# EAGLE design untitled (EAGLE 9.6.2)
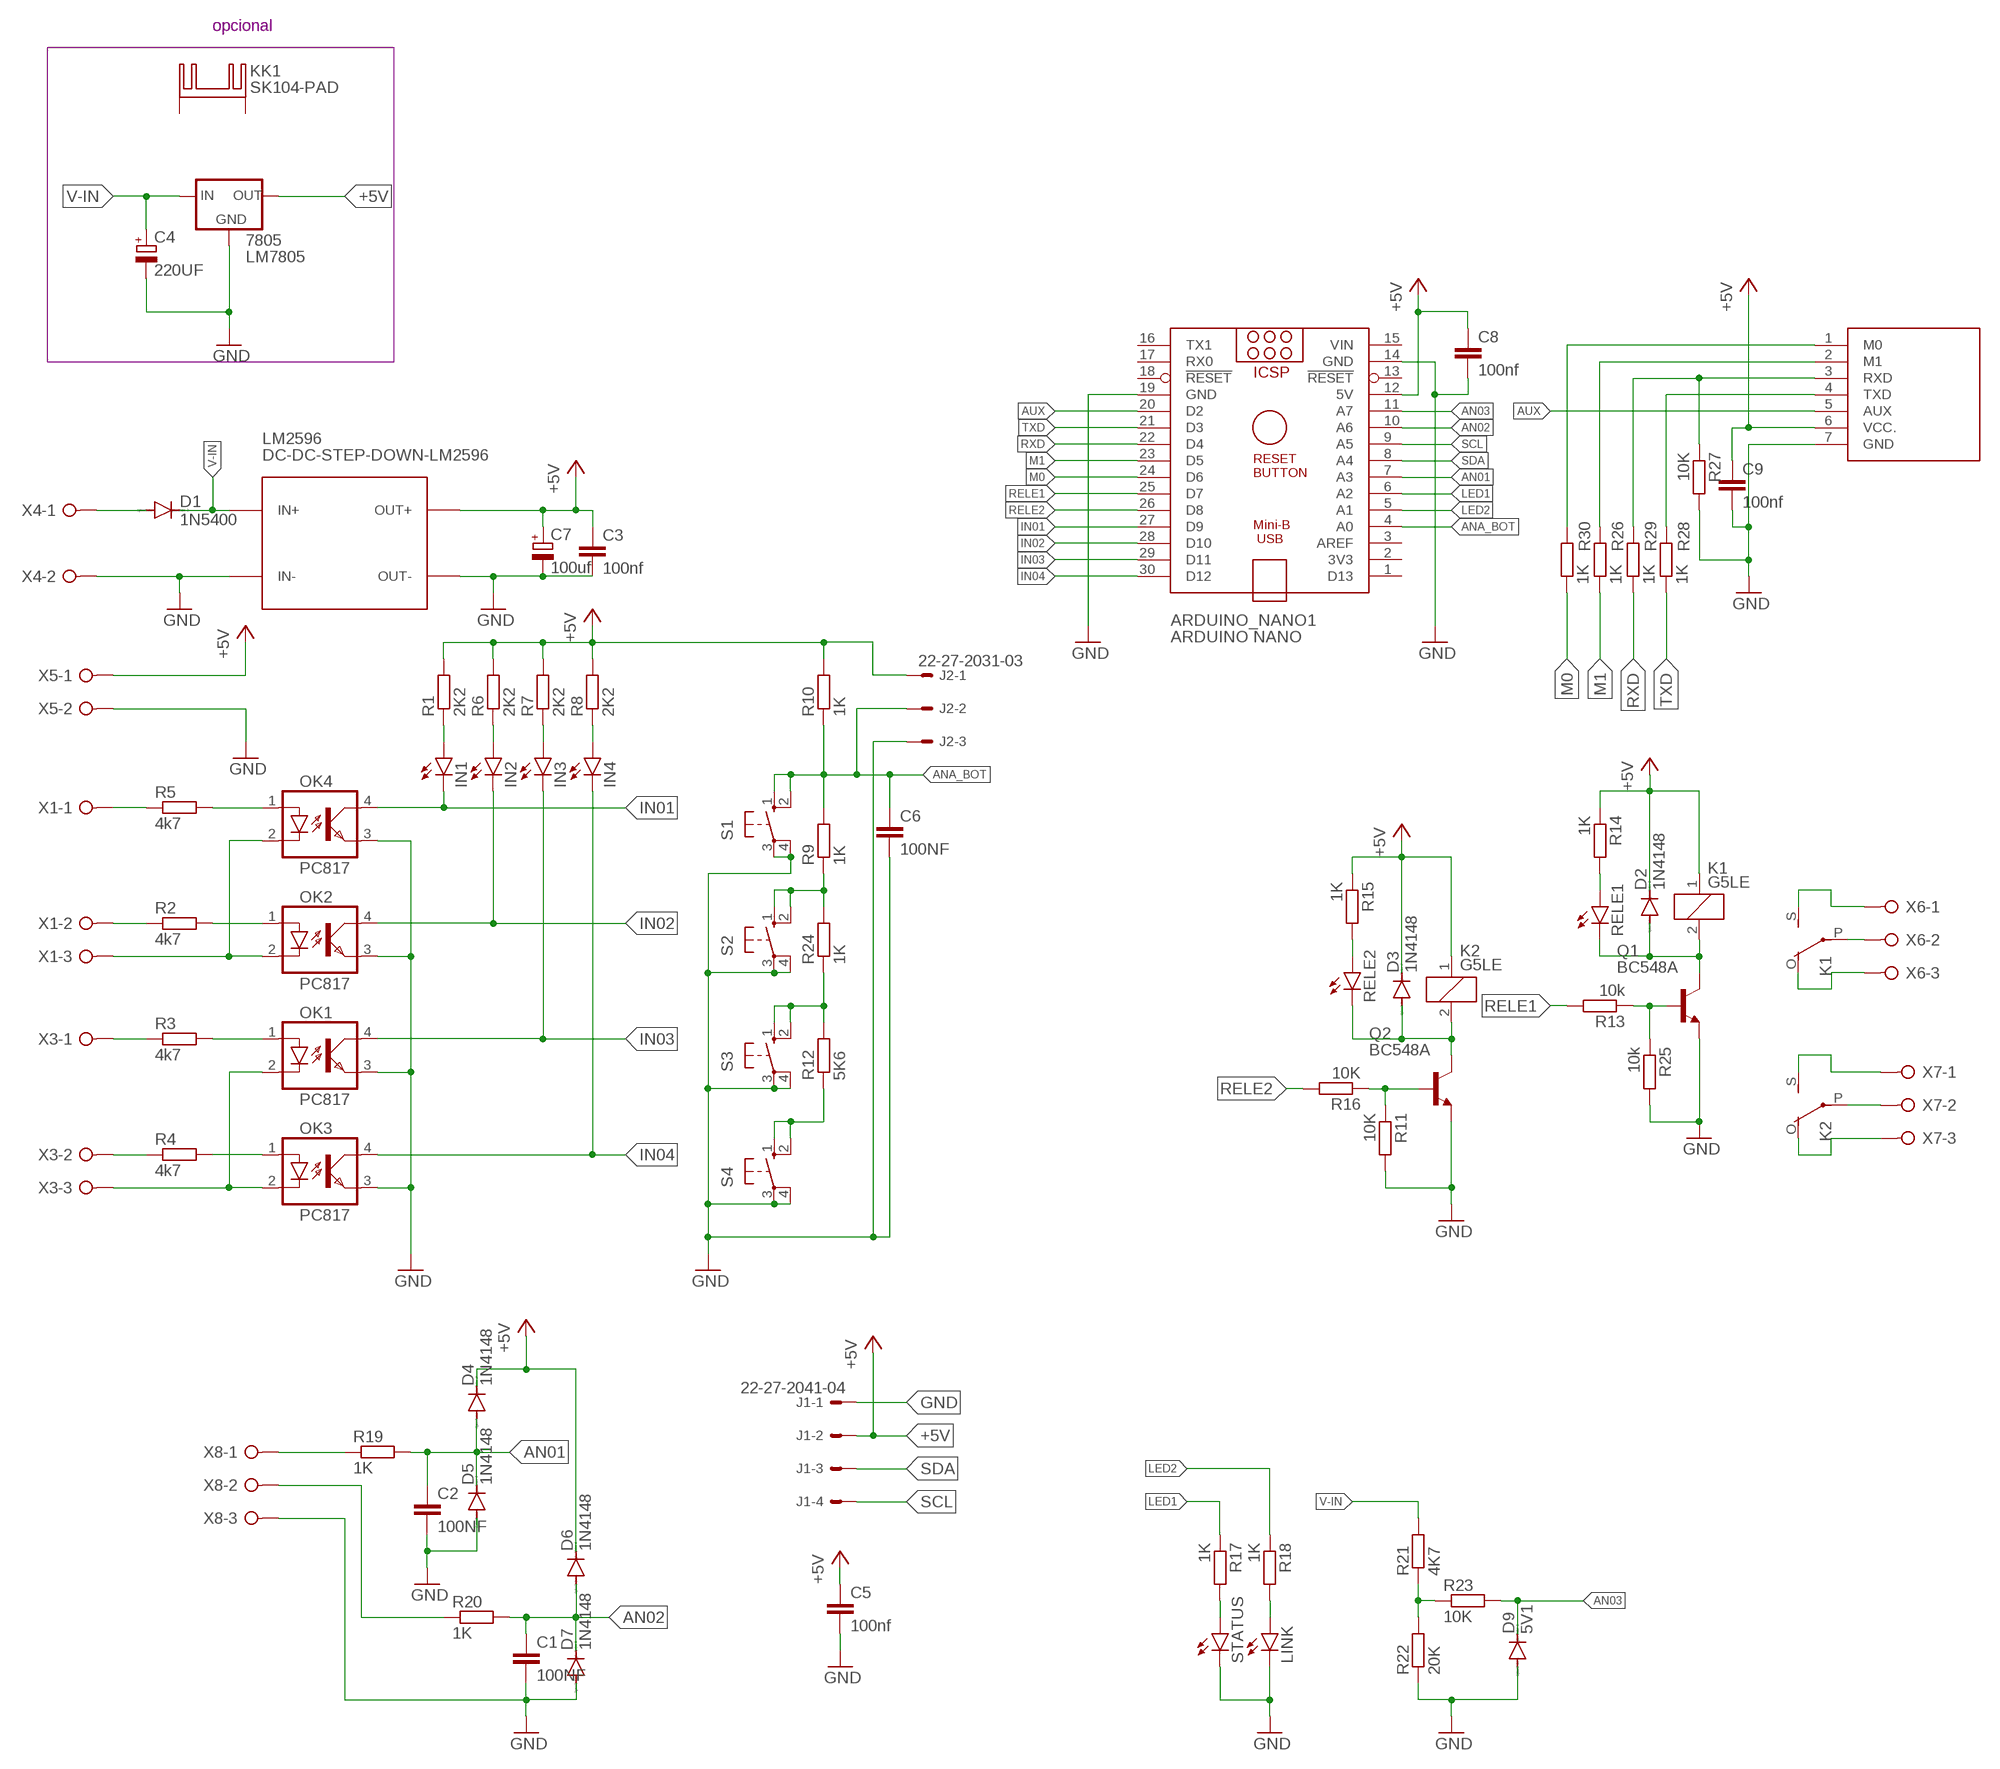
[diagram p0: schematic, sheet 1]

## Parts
7805  LM7805  78XXS  [78XXS]
ARDUINO_NANO1  ARDUINO NANO  ARDUINO_NANO  [ARDUINO_NANO]
C1  100NF  C-EU050-025X075  [C050-025X075]
C2  100NF  C-EU050-025X075  [C050-025X075]
C3  100nf  C-EU025-025X050  [C025-025X050]
C4  220UF  CPOL-EUE5-10.5  [E5-10,5]
C5  100nf  C-EU025-025X050  [C025-025X050]
C6  100NF  C-EU050-025X075  [C050-025X075]
C7  100uf  CPOL-EUE5-10.5  [E5-10,5]
C8  100nf  C-EU025-025X050  [C025-025X050]
C9  100nf  C-EU025-025X050  [C025-025X050]
D1  1N5400  [DO201-15]
D2  1N4148  1N4148DO35-7  [DO35-7]
D3  1N4148  1N4148DO35-7  [DO35-7]
D4  1N4148  1N4148DO35-7  [DO35-7]
D5  1N4148  1N4148DO35-7  [DO35-7]
D6  1N4148  1N4148DO35-7  [DO35-7]
D7  1N4148  1N4148DO35-7  [DO35-7]
D9  5V1  1N4148DO35-7  [DO35-7]
IN1  LED3MM  [LED3MM]
IN2  LED3MM  [LED3MM]
IN3  LED3MM  [LED3MM]
IN4  LED3MM  [LED3MM]
J1  22-27-2041-04  [6410-04]
J2  22-27-2031-03  [6410-03]
K1  G5LE  [G5LE]
K2  G5LE  [G5LE]
KK1  SK104-PAD  [SK104-PAD]
LINK  LED3MM  [LED3MM]
LM2596  DC-DC-STEP-DOWN-LM2596  [DC-DC-STEP-DOWN-LM2596]
OK1  PC817  [DIL04]
OK2  PC817  [DIL04]
OK3  PC817  [DIL04]
OK4  PC817  [DIL04]
Q1  BC548A  [TO92-EBC]
Q2  BC548A  [TO92-EBC]
R1  2K2  R-EU_0204/7  [0204/7]
R2  4k7  R-EU_0204/7  [0204/7]
R3  4k7  R-EU_0204/7  [0204/7]
R4  4k7  R-EU_0204/7  [0204/7]
R5  4k7  R-EU_0204/7  [0204/7]
R6  2K2  R-EU_0204/7  [0204/7]
R7  2K2  R-EU_0204/7  [0204/7]
R8  2K2  R-EU_0204/7  [0204/7]
R9  1K  R-EU_0204/7  [0204/7]
R10  1K  R-EU_0204/7  [0204/7]
R11  10K  R-EU_0204/7  [0204/7]
R12  5K6  R-EU_0204/7  [0204/7]
R13  10k  R-EU_0204/7  [0204/7]
R14  1K  R-EU_0204/7  [0204/7]
R15  1K  R-EU_0204/7  [0204/7]
R16  10K  R-EU_0204/7  [0204/7]
R17  1K  R-EU_0204/7  [0204/7]
R18  1K  R-EU_0204/7  [0204/7]
R19  1K  R-EU_0204/7  [0204/7]
R20  1K  R-EU_0204/7  [0204/7]
R21  4K7  R-EU_0204/7  [0204/7]
R22  20K  R-EU_0204/7  [0204/7]
R23  10K  R-EU_0204/7  [0204/7]
R24  1K  R-EU_0204/7  [0204/7]
R25  10k  R-EU_0204/7  [0204/7]
R26  1K  R-EU_0204/7  [0204/7]
R27  10K  R-EU_0204/7  [0204/7]
R28  1K  R-EU_0204/7  [0204/7]
R29  1K  R-EU_0204/7  [0204/7]
R30  1K  R-EU_0204/7  [0204/7]
RELE1  LED3MM  [LED3MM]
RELE2  LED3MM  [LED3MM]
S1  10-XX  [B3F-10XX]
S2  10-XX  [B3F-10XX]
S3  10-XX  [B3F-10XX]
S4  10-XX  [B3F-10XX]
STATUS  LED3MM  [LED3MM]
U$2  LORAE32  [DIP]
X1  W237-3E  [W237-3E]
X3  W237-3E  [W237-3E]
X4  W237-02P  [W237-132]
X5  W237-02P  [W237-132]
X6  W237-3E  [W237-3E]
X7  W237-3E  [W237-3E]
X8  W237-3E  [W237-3E]

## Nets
+5V: 7805.OUT ARDUINO_NANO1.12(5V) C3.1 C5.1 C7.+ C8.1 C9.1 D2.C D3.C D4.C D6.C J1.2 J2.1 K1.1 K2.1 LM2596.OUT+ R1.2 R6.2 R7.2 R8.2 R10.2 R14.1 R15.1 U$2.6(VCC.) X5.1
AN01: ARDUINO_NANO1.7(A3) C2.1 D4.A D5.C R19.2
AN02: ARDUINO_NANO1.10(A6) C1.1 D6.A D7.C R20.2
AN03: ARDUINO_NANO1.11(A7) D9.C R23.2
ANA_BOT: ARDUINO_NANO1.4(A0) C6.1 J2.2 R9.2 R10.1 S1.1(S) S1.2(S1)
AUX: ARDUINO_NANO1.20(D2) U$2.5(AUX)
BOT03: R12.2 R24.1 S3.1(S) S3.2(S1)
BOT04: R12.1 S4.1(S) S4.2(S1)
GND: 7805.GND ARDUINO_NANO1.14(GND) ARDUINO_NANO1.19(GND) C1.2 C2.2 C3.2 C4.- C5.2 C6.2 C7.- C8.2 C9.2 D5.A D7.A D9.A J1.1 J2.3 LINK.K(C) LM2596.IN- LM2596.OUT- OK1.3(EMIT) OK2.3(EMIT) OK3.3(EMIT) OK4.3(EMIT) Q1.E Q2.E R11.2 R22.1 R25.2 R27.2 S1.3(P) S1.4(P1) S2.3(P) S2.4(P1) S3.3(P) S3.4(P1) S4.3(P) S4.4(P1) STATUS.K(C) U$2.7(GND) X4.2 X5.2 X8.3
IN01: ARDUINO_NANO1.27(D9) IN1.K(C) OK4.4(COL)
IN02: ARDUINO_NANO1.28(D10) IN2.K(C) OK2.4(COL)
IN03: ARDUINO_NANO1.29(D11) IN3.K(C) OK1.4(COL)
IN04: ARDUINO_NANO1.30(D12) IN4.K(C) OK3.4(COL)
LED1: ARDUINO_NANO1.6(A2) R17.1
LED2: ARDUINO_NANO1.5(A1) R18.1
M0: ARDUINO_NANO1.24(D6) R30.1
M1: ARDUINO_NANO1.23(D5) R26.1
N$1: OK1.2(C) OK3.2(C) X3.3
N$2: OK2.2(C) OK4.2(C) X1.3
N$3: OK3.1(A) R4.2
N$4: OK1.1(A) R3.2
N$5: R4.1 X3.2
N$6: R3.1 X3.1
N$7: R5.1 X1.1
N$8: OK4.1(A) R5.2
N$9: R2.1 X1.2
N$10: R27.1 R29.2 U$2.3(RXD)
N$11: D1.A X4.1
N$12: R28.2 U$2.4(TXD)
N$13: OK2.1(A) R2.2
N$14: IN1.A R1.1
N$15: R30.2 U$2.1(M0)
N$16: R26.2 U$2.2(M1)
N$17: IN3.A R7.1
N$18: IN2.A R6.1
N$19: IN4.A R8.1
N$20: K1.S(2:S) X6.1
N$21: K1.O(2:O) X6.3
N$22: K1.P(2:P) X6.2
N$23: K2.P(2:P) X7.2
N$25: K2.S(2:S) X7.1
N$26: R21.1 R22.2 R23.1
N$27: K2.O(2:O) X7.3
N$28: Q1.B R13.1 R25.1
N$29: R19.1 X8.1
N$30: D2.A K1.2 Q1.C RELE1.K(C)
N$31: R14.2 RELE1.A
N$32: D3.A K2.2 Q2.C RELE2.K(C)
N$33: R15.2 RELE2.A
N$34: R20.1 X8.2
N$35: R17.2 STATUS.A
N$36: Q2.B R11.1 R16.1
N$37: LINK.A R18.2
N$40: R9.1 R24.2 S2.1(S) S2.2(S1)
RELE1: ARDUINO_NANO1.25(D7) R13.2
RELE2: ARDUINO_NANO1.26(D8) R16.2
RXD: ARDUINO_NANO1.22(D4) R29.1
SCL: ARDUINO_NANO1.9(A5) J1.4
SDA: ARDUINO_NANO1.8(A4) J1.3
TXD: ARDUINO_NANO1.21(D3) R28.1
V-IN: 7805.IN C4.+ D1.C LM2596.IN+ R21.2
Unconnected: ARDUINO_NANO1.1(D13) ARDUINO_NANO1.2(3V3) ARDUINO_NANO1.3(AREF) ARDUINO_NANO1.13(!RESET) ARDUINO_NANO1.16(TX1) ARDUINO_NANO1.17(RX0) ARDUINO_NANO1.18(!RESET) KK1.K1(K) KK1.K2(K)

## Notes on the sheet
- opcional

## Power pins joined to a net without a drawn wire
VIN: ARDUINO_NANO1.15(VIN)

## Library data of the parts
7805 = v-reg:78XXS: VOLTAGE REGULATOR
ARDUINO_NANO1 = ArduinoNanoV30:ARDUINO_NANO: Arduino Nano V3.0 Overview: The Arduino Nano is a small, complete, and breadboard-friendly board based on the ATmega328 (Arduino Nano 3.x) or ATmega168 (Arduino Nano 2.x). It has more or less the same functionality of the Arduino Duemilanove, but in a different package. It lacks only a DC power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
C1-C3 C5 C6 C8 C9 = rcl:C-EU: CAPACITOR, European symbol; SPICEPREFIX: C
C4 C7 = rcl:CPOL-EU: POLARIZED CAPACITOR, European symbol; SPICEPREFIX: C
D1 = diode:1N5400: DIODE
D2-D7 D9 = diode:1N4148: DIODE
IN1-IN4 LINK RELE1 RELE2 STATUS = led:LED: LED
J1 = con-molex:22-?-04: CONNECTOR wire to board 2.54 mm (.1 inch) pitch header; MF: MOLEX; OC_FARNELL: unknown; OC_NEWARK: unknown
J2 = con-molex:22-?-03: CONNECTOR wire to board 2.54 mm (.1 inch) pitch header; MF: MOLEX; OC_FARNELL: unknown; OC_NEWARK: unknown
K1 K2 = relay:G5LE: RELAY 1 x switch, 10 A/120 V AC, 8 A/30 V DC, Omron; OC_FARNELL: unknown; OC_NEWARK: unknown
KK1 = heatsink:SK104-PAD: HEATSINK
LM2596 = diy-modules:DC-DC-STEP-DOWN-LM2596: DC/DC Step-Down Regulator based on LM2596-ADJ chip
OK1-OK4 = optocoupler:PC817: SHARP OPTO COUPLER; MPN: PC817X4J000F; OC_FARNELL: 9707727; OC_NEWARK: 97K7059
Q1 Q2 = transistor-npn:BC548*: NPN Transistor
R1-R30 = rcl:R-EU_: RESISTOR, European symbol; SPICEPREFIX: R
S1-S4 = switch-omron:10-XX: OMRON SWITCH; MPN: B3F-1000; OC_FARNELL: 176432; OC_NEWARK: 36M3542
U$2 = lora E32:LORAE32
X1 X3 X6-X8 = con-wago-508:W237-3E: WAGO SREW CLAMP; OC_FARNELL: unknown; OC_NEWARK: unknown
X4 X5 = con-wago-508:W237-02P: WAGO SREW CLAMP; OC_FARNELL: unknown; OC_NEWARK: unknown

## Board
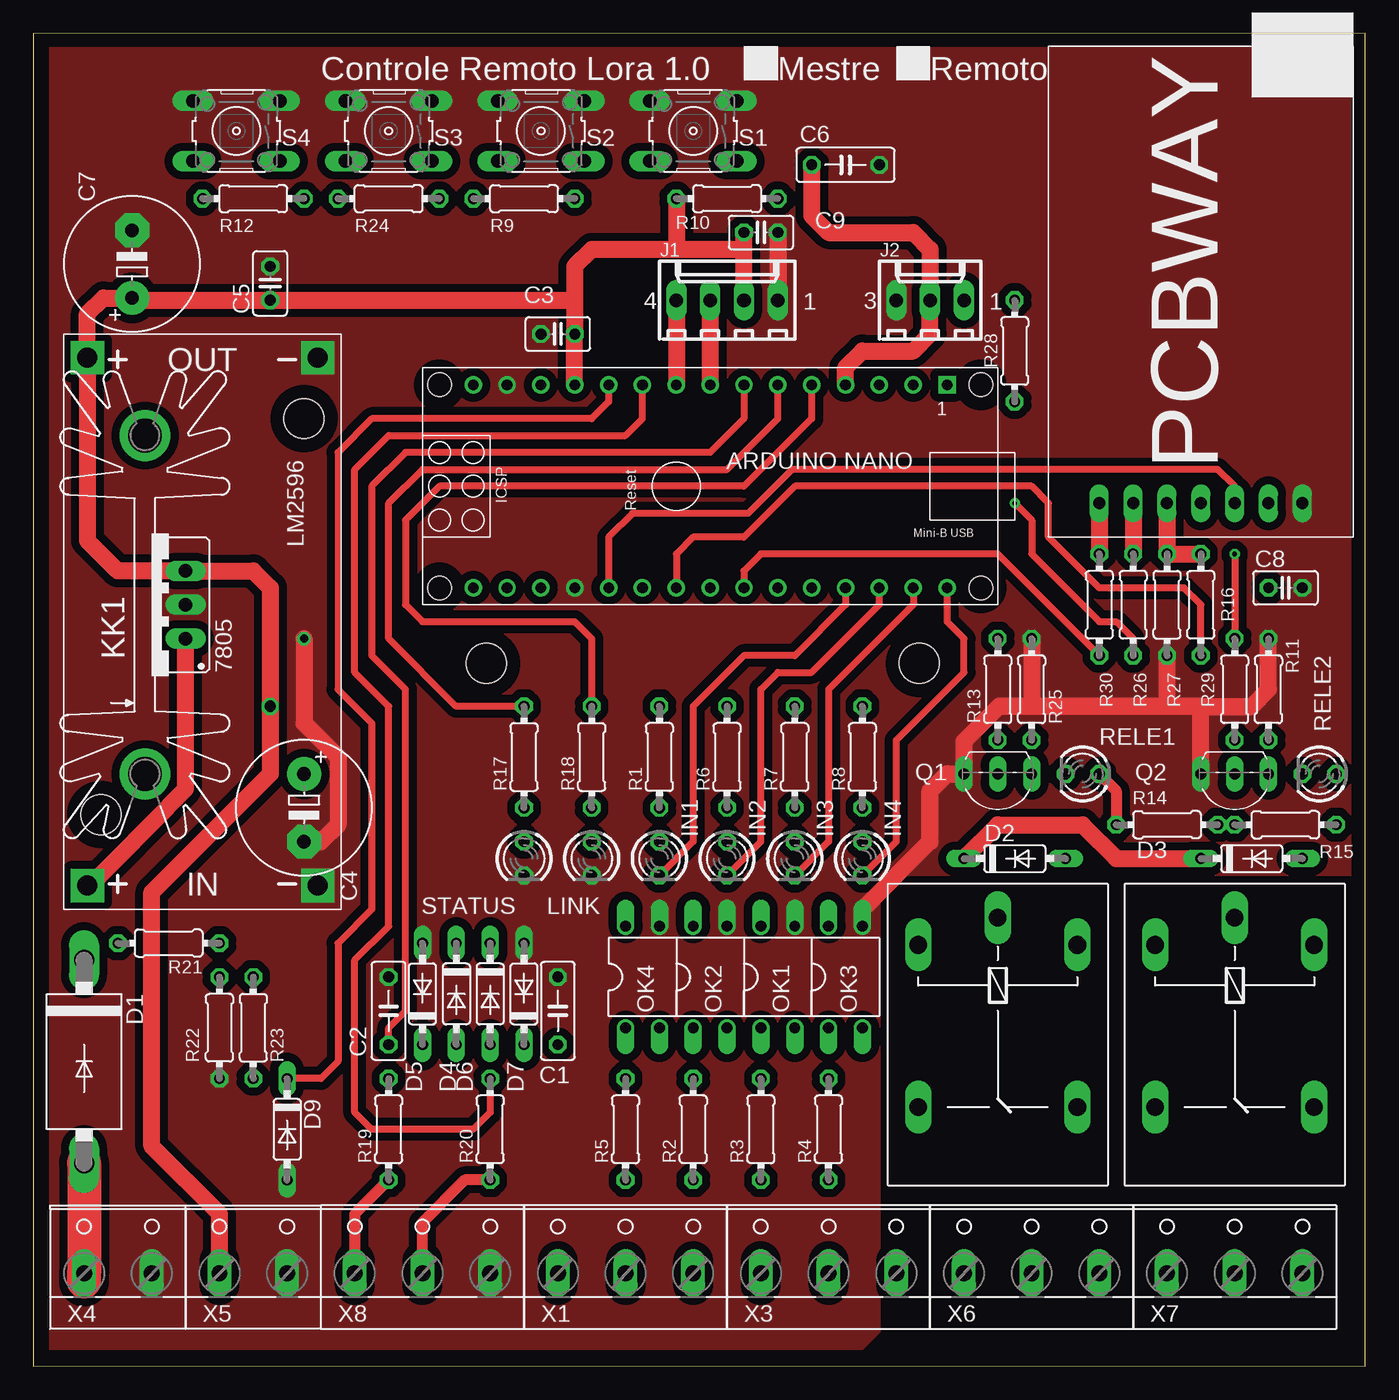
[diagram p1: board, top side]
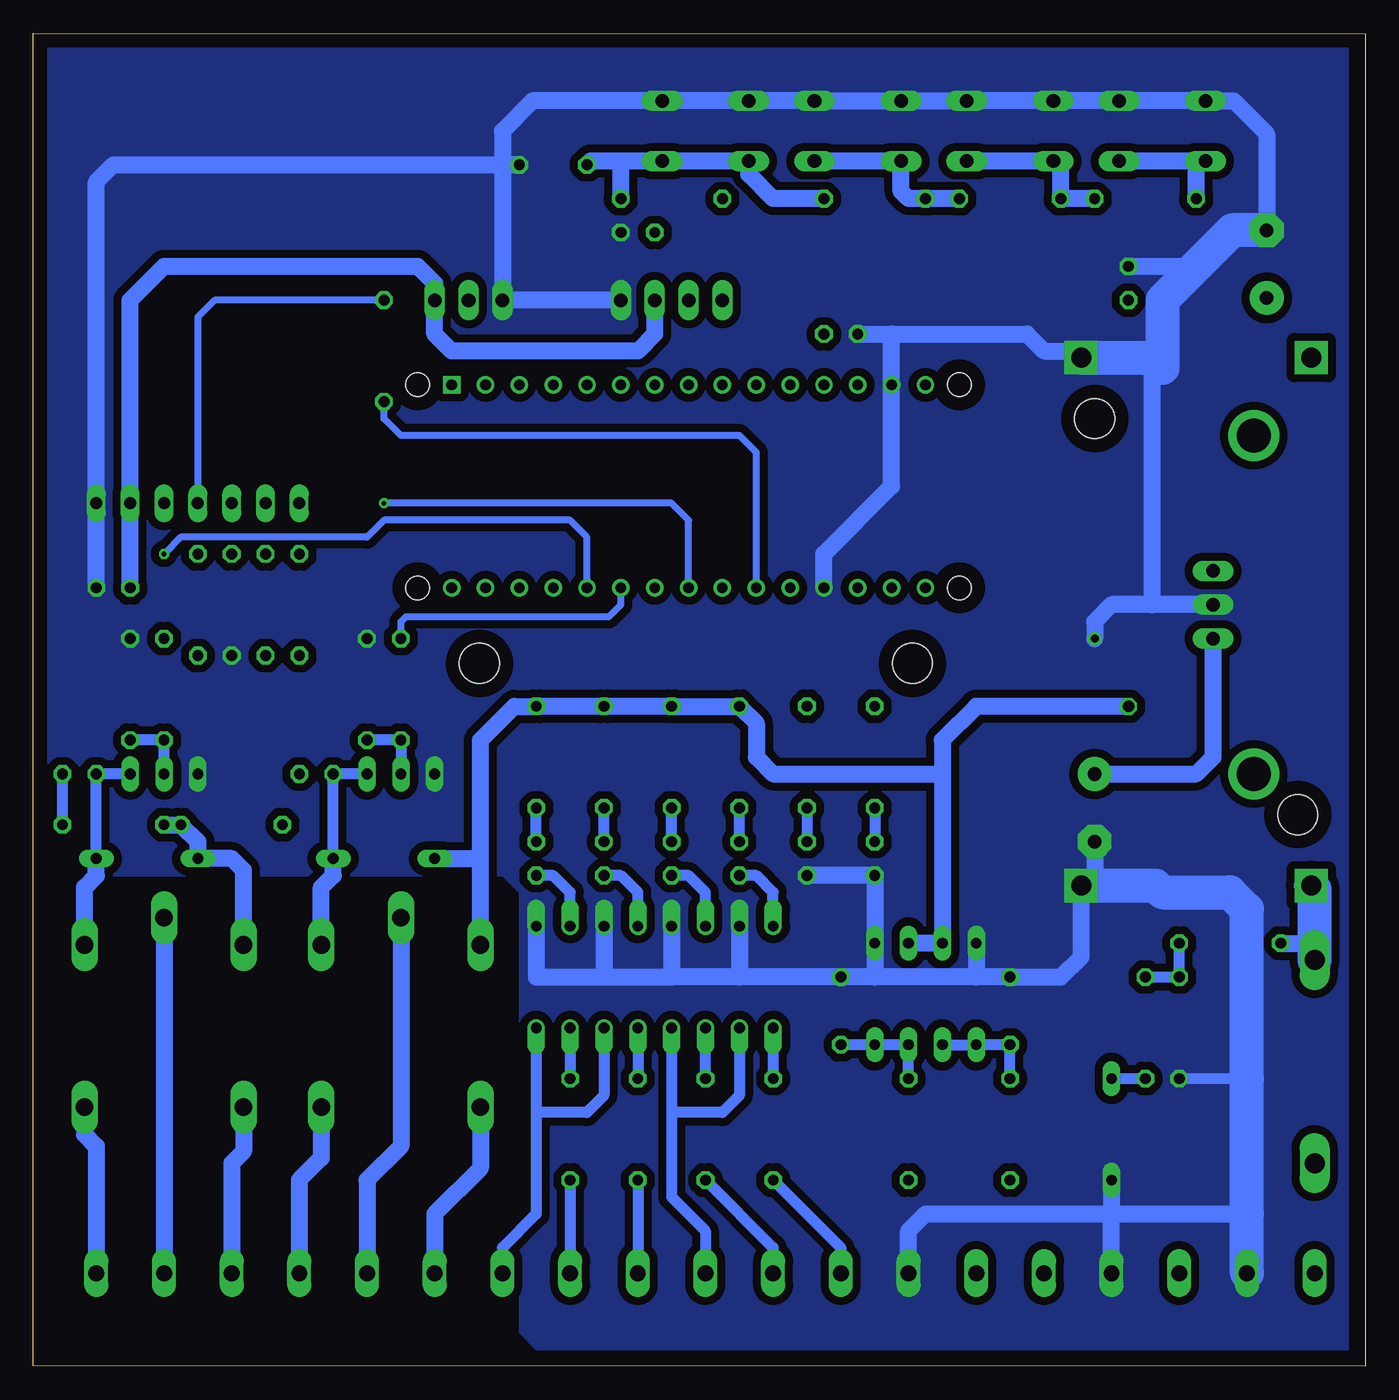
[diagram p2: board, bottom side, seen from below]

Size 99.98 x 100.04 mm. Coordinates in mm from the lower left corner, seen from the top.
Outline: 0,0 99.98,0.04 99.98,100.04 0,100 0,0
Copper layers (1*16): Top 0.035mm / dielectric 1.5mm / Bottom 0.035mm
Design rules "default *": minimum track width 10mil, minimum drill 0.35mm, track to track 10mil, track to pad 10mil, pad to pad 10mil, via to via 10mil, smd to smd 6mil, copper to edge 40mil, drill to drill 6mil, minimum pad ring 10mil, minimum via ring 8mil, stop-mask expansion 4mil, vias tented up to drill 0mil, thermal gap 10mil
Holes 3 mm at 34,52.75 66.5,52.75

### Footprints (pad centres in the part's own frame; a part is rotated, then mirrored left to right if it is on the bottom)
78XXS = drill 1.016 long: GND 0,-2.54; IN -2.54,-2.54; OUT 2.54,-2.54
ARDUINO_NANO = drill 0.8 square: 1 -20.32,-7.62 | drill 0.8: 2 -17.78,-7.62; 3 -15.24,-7.62; 4 -12.7,-7.62; 5 -10.16,-7.62; 6 -7.62,-7.62; 7 -5.08,-7.62; 8 -2.54,-7.62; 9 0,-7.62; 10 2.54,-7.62; 11 5.08,-7.62; 12 7.62,-7.62; 13 10.16,-7.62; 14 12.7,-7.62; 15 15.24,-7.62; 16 15.24,7.62; 17 12.7,7.62; 18 10.16,7.62; 19 7.62,7.62; 20 5.08,7.62; 21 2.54,7.62; 22 0,7.62; 23 -2.54,7.62; 24 -5.08,7.62; 25 -7.62,7.62; 26 -10.16,7.62; 27 -12.7,7.62; 28 -15.24,7.62; 29 -17.78,7.62; 30 -20.32,7.62 | hole 1.778: -22.86,-7.62; -22.86,7.62; 17.78,7.62; 17.78,-7.62
C050-025X075 = drill 0.813 octagon: 1 -2.54,0; 2 2.54,0
C025-025X050 = drill 0.813 octagon: 1 -1.27,0; 2 1.27,0
E5-10,5 = drill 1.016 pad 2.54: + -2.54,0 | drill 1.016 pad 2.54 octagon: - 2.54,0
DO201-15 = drill 1.499 long: A 7.62,0; C -7.62,0
DO35-7 = drill 0.813 long: A 3.81,0; C -3.81,0
LED3MM = drill 0.813 octagon: A -1.27,0; K 1.27,0
6410-04 = drill 1.016 long: 1 3.81,0; 2 1.27,0; 3 -1.27,0; 4 -3.81,0
6410-03 = drill 1.016 long: 1 2.54,0; 2 0,0; 3 -2.54,0
G5LE = drill 1.321 long: 1 -7.493,-5.969; 2 -7.493,5.969; O 4.699,5.969; P -9.525,0; S 4.699,-5.969
SK104-PAD = drill 2.54 pad 3.81: K1 -12.7,-0.762; K2 12.7,-0.762
DC-DC-STEP-DOWN-LM2596 = drill 1.5 pad 2.5 square: IN+ -19.812,8.636; IN- -19.812,-8.636; OUT+ 19.812,8.636; OUT- 19.812,-8.636 | hole 3: -14.478,7.62; 15.24,-7.62
DIL04 = drill 0.813 offset: 1 -1.27,-3.81; 2 1.27,-3.81; 3 1.27,3.81; 4 -1.27,3.81
TO92-EBC = drill 0.813 long: B 0,-1.27; C -2.54,-1.27; E 2.54,-1.27
0204/7 = drill 0.813 octagon: 1 -3.81,0; 2 3.81,0
B3F-10XX = drill 1.016 long: 1 -3.251,2.261; 2 3.251,2.261; 3 -3.251,-2.261; 4 3.251,-2.261
DIP = drill 0.9 long: 1 -3.81,16.51; 2 -3.81,13.97; 3 -3.81,11.43; 4 -3.81,8.89; 5 -3.81,6.35; 6 -3.81,3.81; 7 -3.81,1.27
W237-3E = drill 1.194 long: 1 -5.08,-0.635; 2 0,-0.635; 3 5.08,-0.635
W237-132 = drill 1.194 long: 1 -2.54,-0.635; 2 2.54,-0.635

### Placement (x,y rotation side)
7805  8.89,57.15 90 top
ARDUINO_NANO1  48.26,66.04 180 top
C1  39.37,26.67 90 top
C2  26.67,26.67 90 top
C3  39.37,77.47 180 top
C4  20.32,41.91 270 top
C5  17.78,81.28 90 top
C6  60.96,90.17 0 top
C7  7.41,82.72 90 top
C8  93.98,58.42 0 top
C9  54.61,85.09 0 top
D1  3.81,22.86 270 top
D2  73.66,38.1 0 top
D3  91.44,38.1 0 top
D4  31.75,27.94 270 top
D5  29.21,27.94 90 top
D6  34.29,27.94 270 top
D7  36.83,27.94 90 top
D9  19.05,17.78 270 top
IN1  46.99,38.1 270 top
IN2  52.07,38.1 270 top
IN3  57.15,38.1 270 top
IN4  62.23,38.1 270 top
J1  52.07,80.01 0 top
J2  67.31,80.01 0 top
K1  72.39,24.13 270 top
K2  90.17,24.13 270 top
KK1  7.62,57.15 90 top
LINK  41.91,38.1 270 top
LM2596  12.7,55.88 90 top
OK1  55.88,29.21 0 top
OK2  50.8,29.21 0 top
OK3  60.96,29.21 0 top
OK4  45.72,29.21 0 top
Q1  72.39,43.18 180 top
Q2  90.17,43.18 180 top
R1  46.99,45.72 90 top
R2  49.53,17.78 90 top
R3  54.61,17.78 90 top
R4  59.69,17.78 90 top
R5  44.45,17.78 90 top
R6  52.07,45.72 90 top
R7  57.15,45.72 90 top
R8  62.23,45.72 90 top
R9  36.83,87.63 0 top
R10  52.07,87.63 180 top
R11  92.71,50.8 90 top
R12  16.51,87.63 0 top
R13  72.39,50.8 90 top
R14  85.09,40.64 180 top
R15  93.98,40.64 0 top
R16  90.17,50.8 90 top
R17  36.83,45.72 270 top
R18  41.91,45.72 270 top
R19  26.67,17.78 90 top
R20  34.29,17.78 90 top
R21  10.16,31.75 180 top
R22  13.97,25.4 90 top
R23  16.51,25.4 270 top
R24  26.67,87.63 0 top
R25  74.93,50.8 90 top
R26  82.55,57.15 90 top
R27  85.09,57.15 270 top
R28  73.66,76.2 90 top
R29  87.63,57.15 90 top
R30  80.01,57.15 90 top
RELE1  78.74,44.45 180 top
RELE2  96.52,44.45 180 top
S1  49.53,92.71 180 top
S2  38.1,92.71 180 top
S3  26.67,92.71 180 top
S4  15.24,92.71 180 top
STATUS  36.83,38.1 270 top
U$2  96.52,68.58 90 top
X1  44.45,7.62 0 top
X3  59.69,7.62 0 top
X4  6.35,7.62 0 top
X5  16.51,7.62 0 top
X6  74.93,7.62 0 top
X7  90.17,7.62 0 top
X8  29.21,7.62 0 top

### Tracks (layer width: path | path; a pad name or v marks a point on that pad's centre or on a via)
+5V  (via drill 0.85)
  Top 1.27: J1.2 53.34,83.82 | 53.34,83.82 C9.1 | 53.34,83.82 48.26,83.82 | 48.26,83.82 41.91,83.82 40.64,82.55 40.64,80.01 | 40.64,80.01 C3.1 ARDUINO_NANO1.12 | R10.2 48.26,83.82 | 40.64,80.01 C5.1 7.58,80.01 C7.+ 5.25,80.18 4.06,78.99 LM2596.OUT+ 4.06,61.98 6.35,59.69 7805.OUT 16.51,59.69 17.78,58.42 v17.78,49.53 17.78,44.45 8.89,35.56 8.89,16.51 13.97,11.43 X5.1 | D2.C 72.39,40.64 78.74,40.64 81.28,38.1 D3.C
  Bottom 1.27: U$2.6 C8.1 92.71,80.01 90.17,82.55 71.12,82.55 69.85,81.28 J2.1 69.85,77.47 68.58,76.2 54.61,76.2 53.34,77.47 J1.2 | K1.1 66.42,38.1 | 66.42,38.1 66.42,46.99 63.88,49.53 R8.2 R7.2 R6.2 R1.2 45.72,48.26 45.72,45.72 44.45,44.45 31.75,44.45 | D2.C 66.42,38.1 | D6.C D4.C 31.75,44.45 | K2.1 84.2,37.21 85.09,38.1 D3.C 87.63,39.37 R14.1 R15.1 | v17.78,49.53 29.21,49.53 31.75,46.99 31.75,44.45
AN01
  Top 0.508: ARDUINO_NANO1.7 53.34,71.12 50.8,68.58 27.94,68.58 25.4,66.04 25.4,53.34 27.94,50.8 27.94,26.67 26.67,25.4 C2.1
  Bottom 0.813: D4.A D5.C C2.1 R19.2
AN02
  Top 0.508: R20.2 34.29,19.05 33.02,17.78 25.4,17.78 24.13,19.05 24.13,30.48 26.67,33.02 26.67,49.53 24.13,52.07 24.13,67.31 26.67,69.85 44.45,69.85 45.72,71.12 ARDUINO_NANO1.10
  Bottom 0.813: C1.1 D7.C D6.A R20.2
AN03
  Top 0.508: ARDUINO_NANO1.11 43.18,72.39 41.91,71.12 25.4,71.12 22.86,68.58 22.86,50.8 25.4,48.26 25.4,34.29 22.86,31.75 22.86,22.86 21.59,21.59 D9.C
  Bottom 0.813: D9.C R23.2
ANA_BOT
  Top 1.27: ARDUINO_NANO1.4 60.96,74.93 62.23,76.2 66.04,76.2 67.31,77.47 J2.2 67.31,83.82 66.04,85.09 59.69,85.09 58.42,86.36 C6.1
  Bottom 1.27: R9.2 44.45,87.63 46.28,89.46 S1.2 S1.1 55.88,90.45 | 55.88,90.45 58.14,90.45 C6.1 | R10.1 55.88,90.45
AUX
  Top 0.508: U$2.5 90.17,66.04 88.9,67.31 56.96,67.31 53.66,64.01 44.96,64.01 43.18,62.23 ARDUINO_NANO1.20
BOT03
  Bottom 1.27: R12.2 R24.1 22.86,90.17 23.14,90.17 S3.2 S3.1
BOT04
  Bottom 1.27: S4.2 12.7,90.45 | 12.7,90.45 S4.1 | R12.1 12.7,90.45
GND  (via drill 0.6)
  Top 1.27: C9.2 J1.1 | OK3.3 62.23,34.29 67.31,39.37 67.31,43.18 68.58,44.45 Q1.E 69.85,46.89 72.49,49.53 74.93,49.53 | Q2.E 87.63,49.53 | 87.63,49.53 85.09,49.53 | 85.09,49.53 74.93,49.53 | R25.2 74.93,49.53 | 87.63,49.53 91.44,49.53 92.71,50.8 R11.2 | R27.2 85.09,49.53 | v20.32,54.61 20.32,48.26 22.86,45.72 22.86,40.64 21.59,39.37 C4.-
  Bottom 0.813: R22.1 8.89,21.59
  Bottom 1.27: 19.05,11.43 8.89,11.43 | X5.2 19.05,11.43 | D9.A 19.05,11.43 | X8.3 34.29,10.16 33.02,11.43 19.05,11.43 | LM2596.IN- 21.34,30.73 22.86,29.21 C2.2 29.21,29.21 | C7.- 7.41,92.5 9.88,94.97 S4.4 S4.3 S3.4 S3.3 S2.4 S2.3 S1.4 S1.3 62.51,94.97 64.77,92.71 64.77,90.17 | J1.1 J2.3 64.77,90.17 | 64.77,90.17 C6.2 93.98,90.17 95.25,88.9 U$2.7 C8.2 | C5.2 12.7,82.55 | C3.2 35.56,77.47 | 35.56,77.47 25.4,77.47 24.13,76.2 20.32,76.2 20.83,75.69 LM2596.OUT- | 35.56,77.47 ARDUINO_NANO1.14 35.56,66.04 40.64,60.96 ARDUINO_NANO1.19 | 29.21,29.21 36.83,29.21 | 36.83,29.21 C1.2 46.99,29.21 | 46.99,29.21 52.07,29.21 | 57.15,29.21 62.23,29.21 OK3.3 | 57.15,29.21 52.07,29.21 | OK4.3 46.99,29.21 | OK2.3 52.07,29.21 | OK1.3 57.15,29.21 | 36.83,29.21 D7.A STATUS.K LINK.K | D5.A 29.21,29.21 | 20.07,39.12 C4.- 20.32,36.07 | 16,75.69 16,57.15 7805.GND 19.05,57.15 20.32,55.88 v20.32,54.61
  Bottom 2.54: X4.2 8.89,11.43 8.89,21.59 8.89,34.29 10.16,35.56 15.24,35.56 15.75,36.07 20.32,36.07 LM2596.IN- | LM2596.OUT- 16,75.69 15.24,74.93 15.24,80.01 12.7,82.55 9.99,85.26 C7.-
  pour Top (isolate 0.61, no thermals): 1.27,1.27 1.27,99.06 99.06,99.06 99.06,36.83 64.77,36.83 63.5,35.56 63.5,2.54 62.23,1.27
  pour Bottom (isolate 0.61, no thermals): 1.27,1.27 1.27,99.06 99.06,99.06 99.06,36.83 64.77,36.83 63.5,35.56 63.5,2.54 62.23,1.27
IN01
  Top 0.508: ARDUINO_NANO1.27 60.96,57.15 57.15,53.34 53.34,53.34 49.53,49.53 49.53,39.37 IN1.K
  Bottom 0.813: 44.45,34.29 44.45,35.56 45.72,36.83 IN1.K
  Bottom 1.27: OK4.4 44.45,34.29
IN02
  Top 0.508: IN2.K 54.61,39.37 54.61,50.8 55.88,52.07 58.42,52.07 63.5,57.15 ARDUINO_NANO1.28
  Bottom 0.813: OK2.4 49.53,35.56 50.8,36.83 IN2.K
IN03
  Top 0.508: ARDUINO_NANO1.29 66.04,57.15 59.69,50.8 59.69,39.37 IN3.K
  Bottom 0.813: OK1.4 54.61,35.56 55.88,36.83 IN3.K
IN04
  Top 0.508: IN4.K 64.77,39.37 64.77,46.99 69.85,52.07 69.85,54.61 68.58,55.88 ARDUINO_NANO1.30
  Bottom 0.813: OK3.4 59.69,35.56 60.96,36.83 IN4.K
LED1
  Top 0.508: R17.1 31.75,49.53 26.67,54.61 26.67,64.77 29.21,67.31 52.07,67.31 55.88,71.12 ARDUINO_NANO1.6
LED2
  Top 0.508: ARDUINO_NANO1.5 58.42,71.12 53.34,66.04 30.48,66.04 27.94,63.5 27.94,57.15 29.21,55.88 40.64,55.88 41.91,54.61 R18.1
M0
  Top 0.508: ARDUINO_NANO1.24 53.34,59.69 54.61,60.96 72.39,60.96 R30.1
M1  (via drill 0.35)
  Top 0.508: v73.66,64.77 74.93,63.5 74.93,60.96 80.01,55.88 81.28,55.88 82.55,54.61 R26.1
  Bottom 0.508: ARDUINO_NANO1.23 50.8,63.5 52.07,64.77 v73.66,64.77
N$1
  Bottom 0.813: OK3.2 62.23,19.05 | 62.23,19.05 62.23,11.43 64.77,8.89 X3.3 | OK1.2 57.15,20.32 58.42,19.05 62.23,19.05
N$2
  Bottom 0.813: OK2.2 52.07,19.05 | 52.07,19.05 52.07,12.7 49.53,10.16 X1.3 | OK4.2 46.99,20.32 48.26,19.05 52.07,19.05
N$3
  Bottom 0.813: OK3.1 R4.2
N$4
  Bottom 0.813: OK1.1 R3.2
N$5
  Bottom 0.813: R4.1 X3.2
N$6
  Bottom 0.813: R3.1 X3.1
N$7
  Bottom 0.813: R5.1 39.37,8.89 X1.1
N$8
  Bottom 0.813: OK4.1 R5.2
N$9
  Bottom 0.813: R2.1 44.45,8.89 X1.2
N$10
  Top 1.27: U$2.3 R27.1 R29.2
N$11
  Top 2.54: D1.A X4.1 3.81,6.35
N$12
  Bottom 0.508: R28.2 86.36,80.01 87.63,78.74 U$2.4
N$13
  Bottom 0.813: R2.2 OK2.1
N$14
  Bottom 0.813: IN1.A R1.1
N$15
  Top 1.27: U$2.1 R30.2
N$16
  Top 1.27: U$2.2 R26.2
N$17
  Bottom 0.813: IN3.A R7.1
N$18
  Bottom 0.813: IN2.A R6.1
N$19
  Bottom 0.813: IN4.A R8.1
N$20
  Bottom 1.27: K1.S 66.42,14.86 69.85,11.43 X6.1
N$21
  Bottom 1.27: K1.O 78.36,15.62 80.01,13.97 X6.3
N$22
  Bottom 1.27: K1.P 72.39,16.51 74.93,13.97 X6.2
N$23
  Bottom 1.27: K2.P X7.2
N$25
  Bottom 1.27: K2.S 84.2,16.13 85.09,15.24 X7.1
N$26
  Bottom 0.813: R21.1 R22.2 R23.1
N$27
  Bottom 1.27: K2.O 96.14,17.4 95.25,16.51 X7.3
N$28
  Bottom 0.813: Q1.B R13.1 R25.1
N$29
  Top 0.813: R19.1 24.13,11.43 X8.1
N$30
  Bottom 0.813: D2.A RELE1.K Q1.C
  Bottom 1.27: K1.2 78.36,35.94 77.47,36.83 D2.A
N$31
  Top 0.813: RELE1.A 81.28,43.18 R14.2
N$32
  Bottom 0.813: Q2.C RELE2.K D3.A
  Bottom 1.27: K2.2 96.14,35.94 95.25,36.83 D3.A
N$33
  Bottom 0.813: R15.2 RELE2.A
N$34
  Top 0.813: X8.2 29.21,10.79 32.38,13.97 R20.1
N$35
  Bottom 0.813: R17.2 STATUS.A
N$36
  Bottom 0.813: R11.1 R16.1 Q2.B
N$37
  Bottom 0.813: R18.2 LINK.A
N$40
  Bottom 1.27: R24.2 R9.1 34.29,87.63 34.85,88.19 S2.2 S2.1
RELE1
  Bottom 0.508: R13.2 72.39,55.88 72.01,56.26 56.77,56.26 55.88,57.15 ARDUINO_NANO1.25
RELE2  (via drill 0.35)
  Top 0.508: v90.17,60.96 R16.2
  Bottom 0.508: ARDUINO_NANO1.26 58.42,62.23 59.69,63.5 73.66,63.5 74.93,62.23 88.9,62.23 v90.17,60.96
RXD
  Top 0.508: R29.1 87.63,57.15 86.36,58.42 80.01,58.42 76.2,62.23 76.2,64.77 74.93,66.04 57.15,66.04 53.34,62.23 49.53,62.23 48.26,60.96 ARDUINO_NANO1.22
SCL
  Top 1.27: J1.4 ARDUINO_NANO1.9
SDA
  Top 1.27: J1.3 ARDUINO_NANO1.8
TXD
  Bottom 0.508: ARDUINO_NANO1.21 45.72,68.58 46.99,69.85 72.39,69.85 73.66,71.12 R28.1
V-IN
  Top 1.27: LM2596.IN+ 3.66,35.46 11.43,43.33 7805.IN
  Bottom 1.27: R21.2 3.81,31.75 | C4.+ 12.7,44.45 11.43,45.72 7805.IN
  Bottom 2.54: D1.C 3.81,31.75 3.81,35.81 LM2596.IN+

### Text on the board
tPlace: Controle Remoto Lora 1.0 | Mestre | Remoto | PCBWAY

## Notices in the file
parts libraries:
diy-modules: Released under the Creative Commons Attribution 4.0 International License: http://creativecommons.org/licenses/by/4.0
